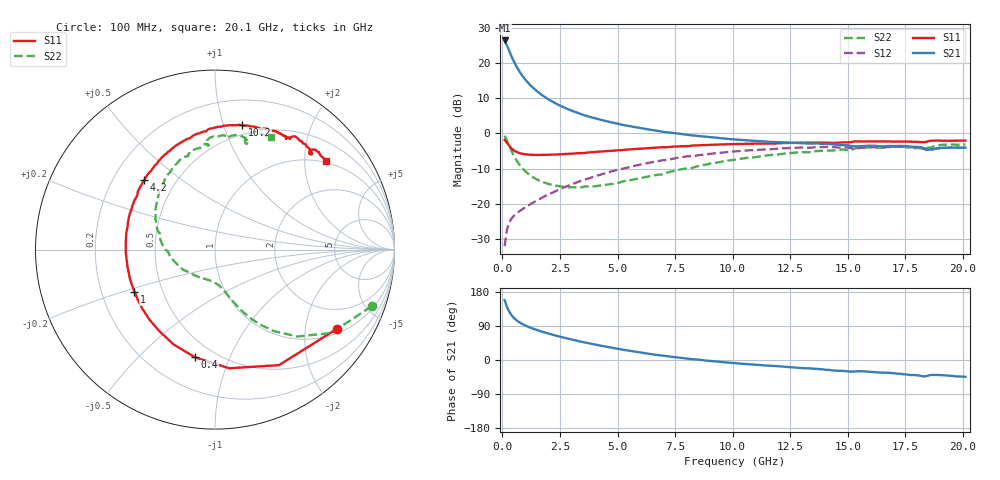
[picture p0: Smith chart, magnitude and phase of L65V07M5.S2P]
!  Infineon Technologies AG
! BFR380L3 , PF131585-7, No.6, Th 09.10.01, soldered on pcb-board, measured with PP GSG850
!  Vce=5.0 V,  Ic=7.5 mA
! Common Emitter S-Parameters:  15. November 2001
#  GHz  S  MA  R  50
! f  S11  S21  S12  S22
! GHz  Mag  Ang  Mag  Ang  Mag  Ang  Mag  Ang
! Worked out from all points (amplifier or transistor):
!   201 points, 100 MHz to 20.1 GHz, reference 50 ohm
!   highest |S21| = 26.3 dB at 100 MHz (marker M1)
!   |S21| within 3 dB of that: start of sweep to 300.6 MHz
!   unconditionally stable (mu >= 1): 2.033 GHz to 4.473 GHz
!   at 3.4 GHz: K = 1.04, MAG = 8.3 dB, |S12| = -13.5 dB
!   at 10.1 GHz: K = 0.93, MSG = 1.7 dB, |S12| = -5.1 dB
!   at 20.1 GHz: K = 0.99, MSG = 0.0 dB, |S12| = -4.0 dB
!   S11 on the Smith chart (normalised r, x): 100 MHz: 1.15, -2.96; 400 MHz: 0.39, -0.75; 1 GHz: 0.35, -0.22; 4.2 GHz: 0.33, +0.37; 10.2 GHz: 0.41, +1.15; 20.1 GHz: 0.95, +2.54
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0.1  0.8097 -33.1  20.74 158.0  0.02535 72.9  0.9278 -19.9
0.2  0.7359 -61.0  17.66 140.4  0.0433 61.4  0.7972 -35.7
0.3  0.6659 -83.2  14.7 127.6  0.05492 53.8  0.6675 -46.5
0.4  0.6105 -100.5  12.32 118.3  0.06247 49.9  0.5628 -54.0
0.5  0.576 -113.7  10.47 111.2  0.06825 47.7  0.4844 -59.2
0.6  0.5497 -124.6  9.045 105.7  0.07308 47.0  0.4247 -63.0
0.7  0.5341 -133.4  7.956 101.1  0.07744 46.8  0.3784 -66.0
0.8  0.5219 -140.7  7.077 97.3  0.08166 47.1  0.3425 -68.3
1  0.5065 -152.4  5.792 91.0  0.09008 48.3  0.2912 -71.9
1.2  0.5005 -161.5  4.895 85.8  0.09868 49.7  0.2569 -75.0
1.4  0.4968 -169.1  4.244 81.2  0.1077 51.0  0.2326 -77.8
1.9  0.4983 176.3  3.194 71.5  0.132 53.4  0.1974 -84.7
2.6  0.5096 161.2  2.396 60.0  0.1681 54.6  0.177 -96.1
3.5  0.5272 145.6  1.841 47.3  0.2185 53.3  0.1742 -111.9
4.2  0.552 135.5  1.583 38.7  0.2576 51.3  0.1821 -127.4
5.2  0.5828 123.2  1.327 27.4  0.3156 46.1  0.2079 -146.3
6.8  0.6318 105.2  1.08 12.5  0.4092 37.2  0.261 -176.7
10.1  0.7088 78.8  0.8198 -8.4  0.5562 15.2  0.4268 138.8
10.2  0.7087 77.8  0.8175 -8.8  0.5588 14.5  0.4311 137.6
13.5  0.7396 60.5  0.7202 -22.9  0.6353 -7.0  0.5543 105.1
16.8  0.7701 48.0  0.6645 -33.8  0.6412 -24.0  0.6446 81.0
20.1  0.7923 38.7  0.6304 -44.4  0.6315 -38.1  0.6986 63.4
